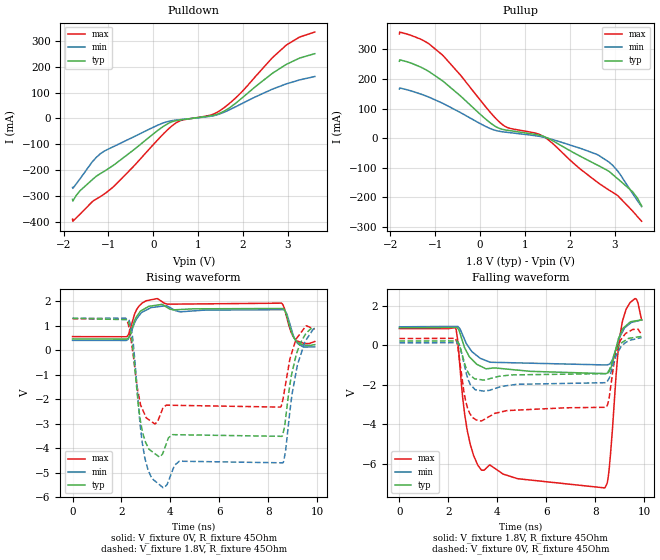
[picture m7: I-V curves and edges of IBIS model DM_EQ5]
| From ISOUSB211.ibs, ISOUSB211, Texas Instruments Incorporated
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[Model]   DM_EQ5
Model_type   Output
Polarity   Inverting
Vmeas = 0.2
Vref = 0
Cref = 15pF
Rref = 45
|   typ   min   max
C_comp   5pF   3pF   8pF
[Voltage Range]   1.8   1.71   1.89
[Temperature Range]   27   150   -40
[Pullup Reference]   1.8   1.71   1.89
[Pulldown Reference]   0   0   0
[Power Clamp Reference]   1.8   1.71   1.89
[GND Clamp Reference]   0   0   0
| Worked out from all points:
|   slope of the pulldown table from 0 to 0.27 V, typ, clamps not added: 7.95 ohm
|   slope of the pullup table from 0 to 0.27 V, typ, clamps not added: 7.94 ohm
|   falling waveform, V_fixture 1.8V, R_fixture 45Ohm: 20-80 % time 292ps typ, 346ps min, 35.9ps max; typ from 0.895 V to 1.3 V
|   rising waveform, V_fixture 0V, R_fixture 45Ohm: 20-80 % time 183ps typ, 189ps min, 104ps max; typ from 0.46 V to 0.225 V
|   rising waveform, V_fixture 1.8V, R_fixture 45Ohm: 20-80 % time 72.6ps typ, 77.1ps min, 75.4ps max; typ from 1.3 V to 0.895 V
|   falling waveform, V_fixture 0V, R_fixture 45Ohm: 20-80 % time 393ps typ, 411ps min, 71.6ps max; typ from 0.225 V to 0.46 V
[Pulldown]
|   Voltage   I(typ)   I(min)   I(max)
-1.8V     -312.3mA   -266.2mA   -388.8mA
-1.795V   -319mA     -269.8mA   -396.8mA
-1.633V   -278.9mA   -232.8mA   -369.2mA
-1.179V   -212.7mA   -136mA     -301.6mA
-865.8mV  -177.8mA   -106.8mA   -260mA
73.8mV    -49.63mA   -27.98mA   -87.09mA
538.2mV   -7.266mA   -5.626mA   -13.71mA
1.294V    10.85mA    9.019mA    13.98mA
1.521V    23.18mA    20.15mA    34.45mA
1.899V    67.71mA    50.57mA    89.7mA
2.947V    206.8mA    132.3mA    280.4mA
3.6V      250.2mA    161.9mA    333.6mA
[Pullup]
|   Voltage   I(typ)   I(min)   I(max)
-1.8V     259.8mA    166.3mA    352.1mA
-1.795V   264.8mA    169.7mA    358.5mA
-1.325V   240.1mA    149.1mA    334.3mA
-849.6mV  194.9mA    118.9mA    282mA
381.6mV   36.3mA     24.84mA    61.51mA
613.8mV   26.64mA    19.55mA    35.63mA
1.402V    6.733mA    3.773mA    6.537mA
2.612V    -90.76mA   -55.24mA   -148.5mA
2.876V    -112.3mA   -81.28mA   -175.5mA
3.065V    -136.9mA   -110.7mA   -193.6mA
3.4V      -181.3mA   -187.3mA   -246.2mA
3.6V      -228.6mA   -231.2mA   -280.5mA
[Ramp]
R_load = 45
|   typ   min   max
dV/dt_r   0.140808/1.48916e-10   0.160407/1.5102e-10   0.120509/1.06682e-10
dV/dt_f   0.243789/2.78937e-10   0.210518/3.16742e-10   0.256824/6.85219e-09
[Falling Waveform]
V_fixture = 1.8V
V_fixture_min = 1.71V
V_fixture_max = 1.89V
R_fixture = 45Ohm
C_fixture = 0F
|   Time   V(typ)   V(min)   V(max)
0s        895mV      947.6mV    856.5mV
2.289ns   917.7mV    968.7mV    911.5mV
2.761ns   -346.3mV   48.61mV    -4.241V
3.348ns   -1.069V    -674.3mV   -6.321V
8.362ns   -1.426V    -986.7mV   -7.224V
8.562ns   -1.337V    -955.5mV   -6.393V
8.917ns   176.2mV    92.66mV    -545.5mV
9.111ns   792.7mV    678.8mV    1.198V
9.63ns    1.243V     1.215V     2.379V
9.9ns     1.301V     1.298V     1.285V
[Rising Waveform]
V_fixture = 0V
V_fixture_min = 0V
V_fixture_max = 0V
R_fixture = 45Ohm
C_fixture = 0F
|   Time   V(typ)   V(min)   V(max)
0s        459.5mV    400.3mV    553.4mV
2.207ns   451.9mV    397.6mV    547.1mV
2.71ns    1.501V     1.397V     1.792V
3.454ns   1.839V     1.768V     2.104V
3.895ns   1.725V     1.786V     1.876V
4.391ns   1.658V     1.566V     1.881V
8.634ns   1.679V     1.653V     1.772V
8.917ns   840.3mV    948.4mV    773.4mV
9.098ns   431.1mV    427.5mV    442.3mV
9.9ns     224.9mV    133mV      352.5mV
[Rising Waveform]
V_fixture = 1.8V
V_fixture_min = 1.71V
V_fixture_max = 1.89V
R_fixture = 45Ohm
C_fixture = 0F
|   Time   V(typ)   V(min)   V(max)
0s        1.301V     1.298V     1.285V
2.314ns   1.071V     1.216V     876.8mV
2.653ns   -1.858V    -1.727V    -1.586V
2.944ns   -3.632V    -4.346V    -2.61V
3.382ns   -4.234V    -5.347V    -3.003V
3.707ns   -4.161V    -5.616V    -2.338V
4.367ns   -3.451V    -4.53V     -2.253V
8.595ns   -3.44V     -4.596V    -2.028V
9.186ns   -52mV      -629.2mV   519.3mV
9.9ns     895mV      947.6mV    856.5mV
[Falling Waveform]
|Gnd
V_fixture = 0V
V_fixture_min = 0V
V_fixture_max = 0V
R_fixture = 45Ohm
C_fixture = 0F
|   Time   V(typ)   V(min)   V(max)
0s        224.9mV    133mV      352.5mV
2.282ns   232.2mV    141.6mV    361.7mV
2.489ns   -139.4mV   -121.4mV   -1.007V
2.774ns   -1.291V    -1.586V    -3.138V
3.337ns   -1.738V    -2.295V    -3.833V
4.388ns   -1.521V    -2.04V     -3.307V
8.434ns   -1.429V    -1.888V    -3.137V
9.027ns   94.43mV    -123.8mV   240.1mV
9.547ns   394.4mV    302.3mV    813.2mV
9.9ns     459.5mV    400.3mV    553.4mV
